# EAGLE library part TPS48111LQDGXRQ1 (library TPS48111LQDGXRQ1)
TPS4811-Q1 100V Automotive Smart High-Side Driver With Protection and Diagnostics , 3.5V ~ 80V , 4A , 19-VSSOP ,-40C ~ 125C (TA) Source: Datasheet
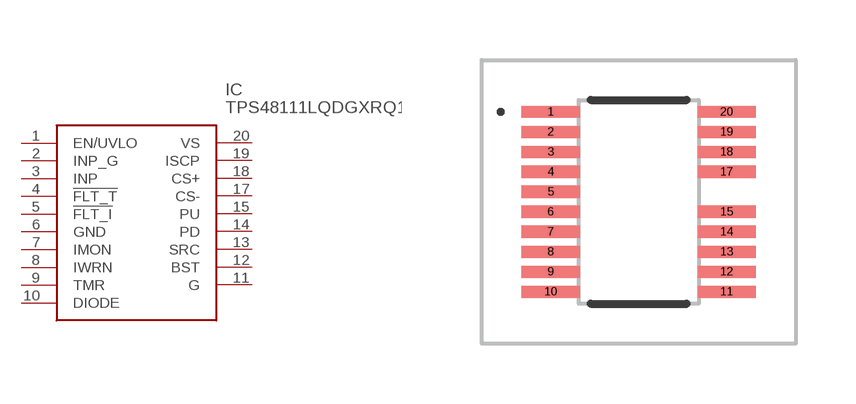
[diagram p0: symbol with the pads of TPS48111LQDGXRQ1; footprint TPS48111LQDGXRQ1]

Designator prefix IC

## TPS48111LQDGXRQ1 (Arrow_Part_Number: TPS48111LQDGXRQ1; Arrow_Price-Stock: https://www.arrow.com/en/products/tps48111lqdgxrq1/texas-instruments.html?utm_currency=USD&region=nac; Description: TPS4811-Q1 100V Automotive Smart High-Side Driver With Protection and Diagnostics , 3.5V ~ 80V , 4A , 19-VSSOP ,-40C ~ 125C (TA); Height: 1.1mm; Manufacturer_Name: Texas Instruments; Manufacturer_Part_Number: TPS48111LQDGXRQ1; Mouser_Part_Number: 595-TPS48111LQDGXRQ1; Mouser_Price-Stock: https://www.mouser.co.uk/ProductDetail/Texas-Instruments/TPS48111LQDGXRQ1?qs=amGC7iS6iy%2Faisrr5sZ5WQ%3D%3D)  [TPS48111LQDGXRQ1]
1  EN/UVLO
2  INP_G
3  INP
4  !FLT_T
5  !FLT_I
6  GND
7  IMON
8  IWRN
9  TMR
10  DIODE
11  G
12  BST
13  SRC
14  PD
15  PU
17  CS-
18  CS+
19  ISCP
20  VS

## Footprint TPS48111LQDGXRQ1 (pad centres in mm)
DGX0019A_2025-20
smd 1.45 x 0.3: 1 -2.2,2.25; 2 -2.2,1.75; 3 -2.2,1.25; 4 -2.2,0.75; 5 -2.2,0.25; 6 -2.2,-0.25; 7 -2.2,-0.75; 8 -2.2,-1.25; 9 -2.2,-1.75; 10 -2.2,-2.25; 11 2.2,-2.25; 12 2.2,-1.75; 13 2.2,-1.25; 14 2.2,-0.75; 15 2.2,-0.25; 17 2.2,0.75; 18 2.2,1.25; 19 2.2,1.75; 20 2.2,2.25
